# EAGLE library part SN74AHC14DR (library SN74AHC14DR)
Hex Schmitt-Trigger Inverters Source: Datasheet
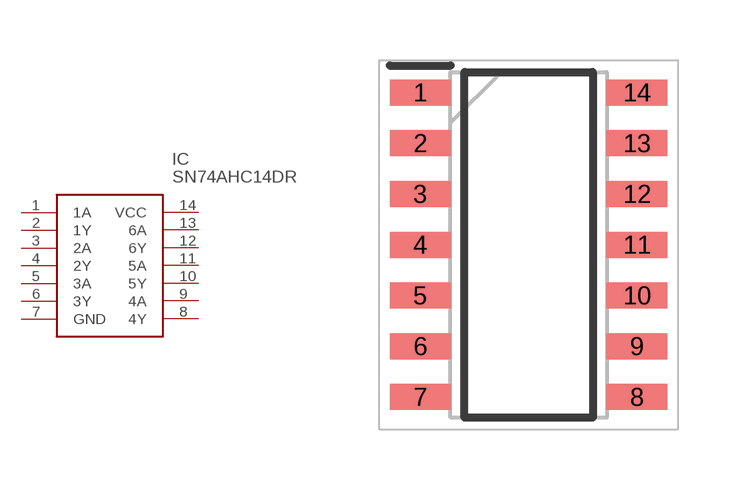
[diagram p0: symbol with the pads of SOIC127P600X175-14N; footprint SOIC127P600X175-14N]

Designator prefix IC

## SN74AHC14DR (Description: Hex Schmitt-Trigger Inverters; Height: 1.75mm; Manufacturer_Name: Texas Instruments; Manufacturer_Part_Number: SN74AHC14DR; Mouser_Part_Number: 595-SN74AHC14DR; Mouser_Price-Stock: https://www.mouser.co.uk/ProductDetail/Texas-Instruments/SN74AHC14DR?qs=ZA235jQDfbrd%252BwhwnzLskw%3D%3D)  [SOIC127P600X175-14N]
1  1A
2  1Y
3  2A
4  2Y
5  3A
6  3Y
7  GND
8  4Y
9  4A
10  5Y
11  5A
12  6Y
13  6A
14  VCC

## Footprint SOIC127P600X175-14N (pad centres in mm)
D (-R-PDSO-G14)
smd 1.525 x 0.65: 1 -2.712,3.81; 2 -2.712,2.54; 3 -2.712,1.27; 4 -2.712,0; 5 -2.712,-1.27; 6 -2.712,-2.54; 7 -2.712,-3.81; 8 2.712,-3.81; 9 2.712,-2.54; 10 2.712,-1.27; 11 2.712,0; 12 2.712,1.27; 13 2.712,2.54; 14 2.712,3.81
